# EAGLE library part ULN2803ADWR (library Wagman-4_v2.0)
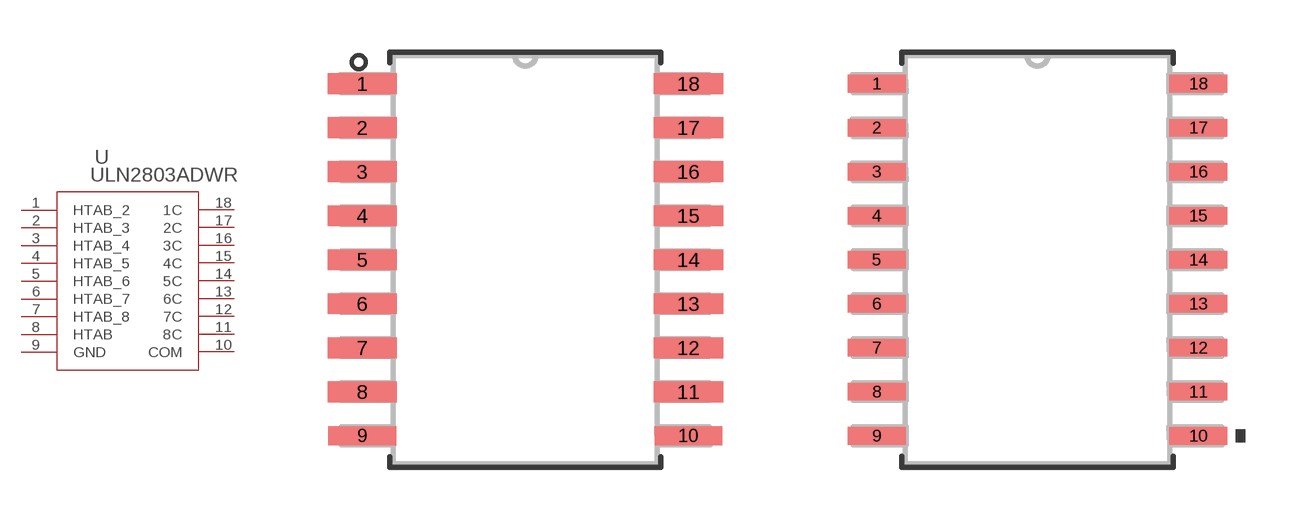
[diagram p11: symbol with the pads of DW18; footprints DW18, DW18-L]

Designator prefix U

## ULN2803ADWR (MANUFACTURER_PART_NUMBER: ULN2803ADWR; VENDOR: Texas Instruments)  [DW18]
1  HTAB_2  pwr
2  HTAB_3  pwr
3  HTAB_4  pwr
4  HTAB_5  pwr
5  HTAB_6  pwr
6  HTAB_7  pwr
7  HTAB_8  pwr
8  HTAB  pwr
9  GND  pwr
10  COM  pas
11  8C  out
12  7C  out
13  6C  out
14  5C  out
15  4C  out
16  3C  out
17  2C  out
18  1C  out

## ULN2803ADWRDW18-L (MANUFACTURER_PART_NUMBER: ULN2803ADWR; VENDOR: Texas Instruments)  [DW18-L]
Pads as for DW18

## ULN2803ADWRDW18-M (MANUFACTURER_PART_NUMBER: ULN2803ADWR; VENDOR: Texas Instruments)  [DW18-M]
Pads as for DW18

## Footprint DW18 (pad centres in mm)
smd 2 x 0.6: 1 -4.7,5.08; 2 -4.7,3.81; 3 -4.7,2.54; 4 -4.7,1.27; 5 -4.7,0; 6 -4.7,-1.27; 7 -4.7,-2.54; 8 -4.7,-3.81; 11 4.7,-3.81; 12 4.7,-2.54; 13 4.7,-1.27; 14 4.7,0; 15 4.7,1.27; 16 4.7,2.54; 17 4.7,3.81; 18 4.7,5.08
smd 1.95 x 0.55: 9 -4.7,-5.08; 10 4.7,-5.08

## Footprint DW18-L (pad centres in mm)
smd 1.676 x 0.508: 1 -4.636,5.08; 2 -4.636,3.81; 3 -4.636,2.54; 4 -4.636,1.27; 5 -4.636,0; 6 -4.636,-1.27; 7 -4.636,-2.54; 8 -4.636,-3.81; 9 -4.636,-5.08; 10 4.636,-5.08; 11 4.636,-3.81; 12 4.636,-2.54; 13 4.636,-1.27; 14 4.636,0; 15 4.636,1.27; 16 4.636,2.54; 17 4.636,3.81; 18 4.636,5.08

## Footprint DW18-M (pad centres in mm)
smd 2.286 x 0.61: 1 -4.737,5.08; 2 -4.737,3.81; 3 -4.737,2.54; 4 -4.737,1.27; 5 -4.737,0; 6 -4.737,-1.27; 7 -4.737,-2.54; 8 -4.737,-3.81; 9 -4.737,-5.08; 10 4.737,-5.08; 11 4.737,-3.81; 12 4.737,-2.54; 13 4.737,-1.27; 14 4.737,0; 15 4.737,1.27; 16 4.737,2.54; 17 4.737,3.81; 18 4.737,5.08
